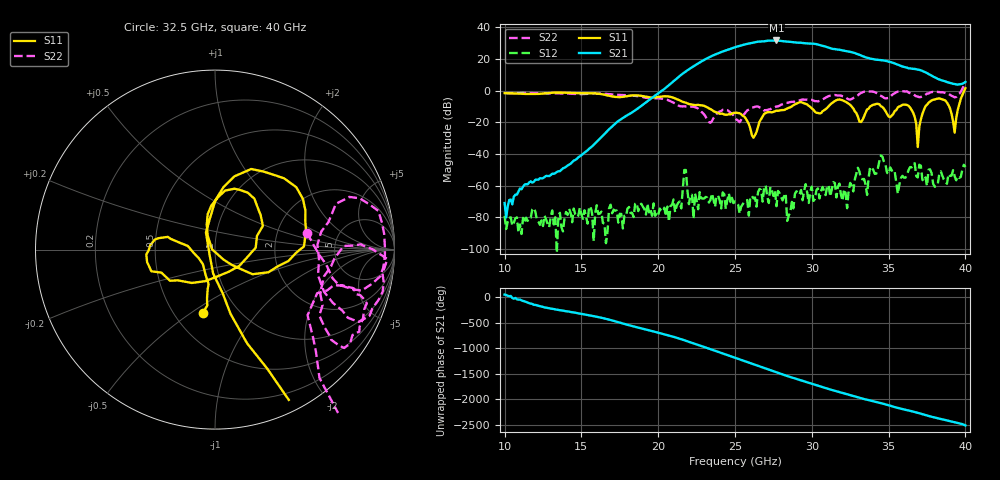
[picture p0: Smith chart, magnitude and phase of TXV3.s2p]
!Keysight Technologies,M9808A,MY58100618,A.14.70.03
!Date: Monday, February 27, 2023 13:18:57
!Correction: S11(C  2-Port  )
!S21(C  2-Port  )
!S12(C  2-Port  )
!S22(C  2-Port  )
!S2P File: Measurements: S11, S21, S12, S22:
# Hz S  RI  R 50
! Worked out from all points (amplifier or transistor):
!   301 points, 10 GHz to 40 GHz, reference 50 ohm
!   highest |S21| = 31.8 dB at 27.7 GHz (marker M1)
!   |S21| within 3 dB of that: 25.44 GHz to 30.54 GHz (5.106 GHz wide, 18.2 % of centre)
!   unconditionally stable (mu >= 1): start of sweep to 39.74 GHz
!   at 15 GHz: K = 52191.67, MAG = -31.5 dB, |S12| = -78.2 dB
!   at 25 GHz: K = 62.06, MAG = 27.8 dB, |S12| = -69.9 dB
!   at 40 GHz: K = 63.09, MSG = 26.9 dB, |S12| = -48.1 dB
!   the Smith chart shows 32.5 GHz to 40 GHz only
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1e10  0.7155 0.4398  0.000159 0.000235  2.49e-05 0.000109  0.0496 0.8406
1.5e10  0.6436 -0.5295  0.00742 0.0054  -0.000123 7.95e-06  0.7539 0.2103
2e10  -0.2059 -0.598  0.7292 0.374  7.99e-05 -8.43e-05  0.2406 -0.5254
2.26e10  -0.3418 -0.104  -6.206 3.853  0.000167 -6.77e-05  0.00902 -0.2714
2.34e10  -0.2536 -0.0713  5.214 10.72  0.000269 -0.000229  -0.0607 -0.0757
2.42e10  -0.1803 0.0496  16.22 -6.243  0.000602 -0.00012  -0.2242 -0.1094
2.5e10  -0.1417 0.1409  -6.068 -22.97  0.000319 1.55e-05  -0.1211 -0.071
2.58e10  -0.0626 0.0895  -29.87 5.188  0.000311 -0.000166  -0.1692 0.1695
2.65e10  0.0716 -0.000548  -3.125 35.35  -0.000436 0.00046  -0.2265 0.2195
2.72e10  0.1892 -0.0943  35.89 13.63  0.000227 0.000169  -0.1047 0.2344
2.77e10  0.1849 -0.1458  32.52 -21.14  0.000148 -0.000169  0.0246 0.3176
2.82e10  0.112 -0.2197  3.909 -36.48  -0.000409 -0.000236  0.0676 0.3811
2.89e10  0.0476 -0.3692  -29.44 -16.29  -0.000436 -0.000349  0.1328 0.4378
2.94e10  0.07 -0.4129  -30.72 9.71  -0.000246 -0.000243  0.1469 0.5052
3e10  0.0839 -0.266  -8.481 29.68  -0.000928 -9.83e-05  0.2337 0.4586
3.08e10  -0.1943 -0.1459  22.76 11.63  -0.00067 7.25e-05  0.5012 0.2618
3.19e10  -0.2715 -0.4379  7.962 -17.6  -0.000124 0.000501  0.5871 0.3792
3.3e10  -0.0517 -0.1436  -13.57 -4.321  0.000915 -0.00358  0.6885 -0.1955
3.4e10  -0.361 0.0243  -5.329 8.444  0.0012 0.00294  0.9101 0.2157
3.5e10  0.00198 -0.1542  6.1 5.575  0.00175 0.00152  0.5741 -0.1443
3.65e10  -0.0208 0.2446  1.301 -4.82  -0.00302 0.00228  0.8118 0.0297
4e10  0.5435 -1.068  1.897 0.211  -0.00292 -0.00262  1.07 -1.444
